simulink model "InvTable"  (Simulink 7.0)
settings: Solver=FixedStepDiscrete  StartTime=0.0  StopTime=inf  FixedStep=samplePeriod  RelTol=1e-3
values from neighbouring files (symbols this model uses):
  forceCanon = 0.00444822    [initialize.m]    (also in TableInit.m = 1)
  iactParams = [	actParams    [initialize.m]
  inertia = inertia + inertiaP2Q([0 0 0], massA(i), cgA(:,i)-cg,  									inertiaCanon, massCanon)    [initialize.m]    (also in TableInit.m = [Ixx 0 0; 0 Iyy 0; 0 0 Izz])
  inertiaMask = zeros(3, 1)    [initialize.m]
  initDispl = zeros(6, 1)    [initialize.m]
  lengthCanon = 25.4    [initialize.m]    (also in TableInit.m)
  mass = ones(3, 1) * (sum(massA) + massT + massS)    [initialize.m]    (also in TableInit.m = 17300)
  massMask = zeros(3, 1)    [initialize.m]
  returnPress = 50    [initialize.m]    (also in TableInit.m)
  rtg = cg    [initialize.m]    (also in TableInit.m = [0 0 cg])
  staticForce = forceT2A(ftbl, dtbl0, dof, rh, rb, rl, canon, atype)    [initialize.m]
undefined symbols (not defined in the file or in its folder): atype, friction, yieldDispl
libraries: LibTransforms x15, LibDynamics x12

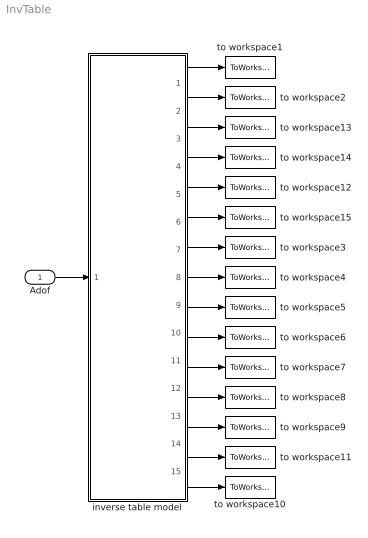
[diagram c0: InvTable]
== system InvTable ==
  Adof : Inport  PortDimensions=6  OutDataType=sfix(16)  OutScaling=2^0
  inverse table model : Subsystem
  to workspace1 : ToWorkspace  VariableName=xyz  SampleTime=-1  SaveFormat=Array
  to workspace10 : ToWorkspace  VariableName=svcmd  SampleTime=-1  SaveFormat=Array
  to workspace11 : ToWorkspace  VariableName=press  SampleTime=-1  SaveFormat=Array
  to workspace12 : ToWorkspace  VariableName=Axyz  SampleTime=-1  SaveFormat=Array
  to workspace13 : ToWorkspace  VariableName=Vxyz  SampleTime=-1  SaveFormat=Array
  to workspace14 : ToWorkspace  VariableName=Vrpw  SampleTime=-1  SaveFormat=Array
  to workspace15 : ToWorkspace  VariableName=Arpw  SampleTime=-1  SaveFormat=Array
  to workspace2 : ToWorkspace  VariableName=rpw  SampleTime=-1  SaveFormat=Array
  to workspace3 : ToWorkspace  VariableName=Fxyz  SampleTime=-1  SaveFormat=Array
  to workspace4 : ToWorkspace  VariableName=Frpw  SampleTime=-1  SaveFormat=Array
  to workspace5 : ToWorkspace  VariableName=Dact  SampleTime=-1  SaveFormat=Array
  to workspace6 : ToWorkspace  VariableName=Vact  SampleTime=-1  SaveFormat=Array
  to workspace7 : ToWorkspace  VariableName=Aact  SampleTime=-1  SaveFormat=Array
  to workspace8 : ToWorkspace  VariableName=Fact  SampleTime=-1  SaveFormat=Array
  to workspace9 : ToWorkspace  VariableName=flow  SampleTime=-1  SaveFormat=Array
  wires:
  inverse table model/1(xyz) -> to workspace1/1
  inverse table model/2(rpw) -> to workspace2/1
  inverse table model/7(Fxyz) -> to workspace3/1
  inverse table model/8(Frpw) -> to workspace4/1
  inverse table model/9(Dact) -> to workspace5/1
  inverse table model/10(Vact) -> to workspace6/1
  inverse table model/11(Aact) -> to workspace7/1
  inverse table model/12(Fact) -> to workspace8/1
  inverse table model/13(flow) -> to workspace9/1
  inverse table model/14(press) -> to workspace11/1
  Adof/1 -> inverse table model/1(Adof)
  inverse table model/15(svcmd) -> to workspace10/1
  inverse table model/3(Vxyz) -> to workspace13/1
  inverse table model/4(Vrpw) -> to workspace14/1
  inverse table model/5(Axyz) -> to workspace12/1
  inverse table model/6(Arpw) -> to workspace15/1

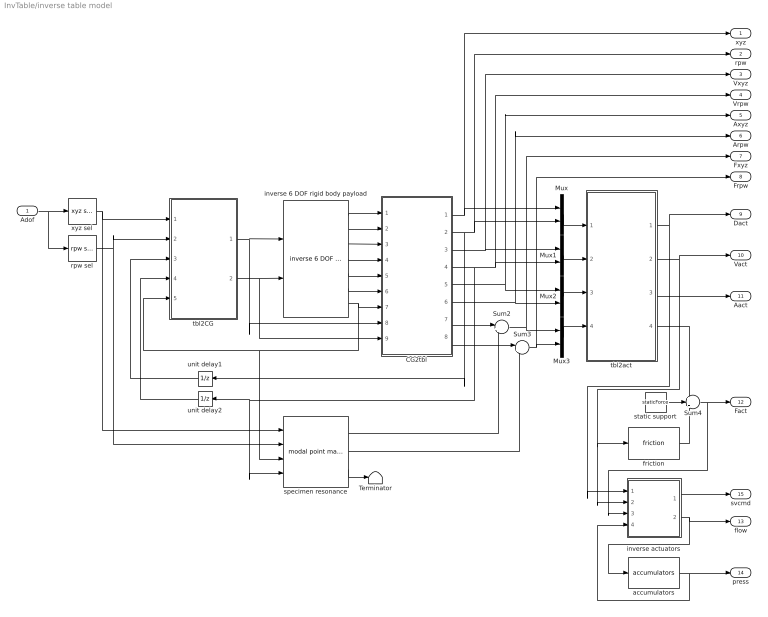
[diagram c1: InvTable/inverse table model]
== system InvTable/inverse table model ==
  Adof : Inport  PortDimensions=6  OutDataType=sfix(16)  OutScaling=2^0
  CG2tbl : Subsystem  mask{ofst=-rtg}
      mask prompts: ofst "Origin offset"
  Mux{,1..3} (4 alike) : Mux  Inputs=2
  Sum2 : Sum  Inputs=|++  OutDataType=sfix(16)  OutScaling=2^0
  Sum3 : Sum  Inputs=|++  OutDataType=sfix(16)  OutScaling=2^0
  Sum4 : Sum  Inputs=+-+  OutDataType=sfix(16)  OutScaling=2^0
  Terminator : Terminator
  accumulators : LibDynamics/accumulators  SystemSampleTime=-1  pumpFlow=pumpFlow  supplyPressure=supplyPress  precharge=precharge  bottleVolume=volume  gasConstant=gasConstant  flowCanon=flowCanon  volumeCanon=volumeCanon  samplePeriod=samplePeriod
  friction : LibDynamics/friction  SystemSampleTime=-1  friction=friction * forceCanon  yieldDispl=yieldDispl * lengthCanon  hysteresis=0  velocCanon=linVelocCanon  samplePeriod=samplePeriod
  inverse 6 DOF rigid body payload : LibDynamics/inverse 6 DOF rigid body payload  SystemSampleTime=-1  mass=mass.*massMask  inertia=diag(inertia.*inertiaMask)  gee=gee  massCanon=massCanon  inertiaCanon=inertiaCanon  linVelocCanon=linVelocCanon  linAccelCanon=linAccelCanon  rotDisplCanon=rotDisplCanon  rotVelocCanon=rotVelocCanon  rotAccelCanon=rotAccelCanon  rotForceCanon=rotForceCanon  initialPosition=initDispl  samplePeriod=samplePeriod
  inverse actuators : Subsystem
  rpw sel : LibTransforms/rpw sel  SystemSampleTime=-1  dof=1:6
  specimen resonance : LibDynamics/modal point mass  SystemSampleTime=-1  mass=modalMass  freq=modalFreq  damp=modalDamp  ofst=modalCG  gee=gee  massCanon=massCanon  linAccelCanon=linAccelCanon  rotDisplCanon=rotDisplCanon  rotVelocCanon=rotVelocCanon  rotForceCanon=rotForceCanon  samplePeriod=samplePeriod
  static support : Constant  Value=staticForce  OutDataType=sfix(16)  OutScaling=2^0
  tbl2CG : Subsystem  mask{ofst=rtg}
      mask prompts: ofst "Origin offset"
  tbl2act : Subsystem
  unit delay1 : UnitDelay  Orientation=left  X0=initDispl(4:6)  SampleTime=-1
  unit delay2 : UnitDelay  Orientation=left  SampleTime=-1
  xyz sel : LibTransforms/xyz sel  SystemSampleTime=-1  dof=1:6
  xyz : Outport  OutDataType=sfix(16)  OutScaling=2^0
  rpw : Outport  Port=2  OutDataType=sfix(16)  OutScaling=2^0
  Vxyz : Outport  Port=3  OutDataType=sfix(16)  OutScaling=2^0
  Vrpw : Outport  Port=4  OutDataType=sfix(16)  OutScaling=2^0
  Axyz : Outport  Port=5  OutDataType=sfix(16)  OutScaling=2^0
  Arpw : Outport  Port=6  OutDataType=sfix(16)  OutScaling=2^0
  Fxyz : Outport  Port=7  OutDataType=sfix(16)  OutScaling=2^0
  Frpw : Outport  Port=8  OutDataType=sfix(16)  OutScaling=2^0
  Dact : Outport  Port=9  OutDataType=sfix(16)  OutScaling=2^0
  Vact : Outport  Port=10  OutDataType=sfix(16)  OutScaling=2^0
  Aact : Outport  Port=11  OutDataType=sfix(16)  OutScaling=2^0
  Fact : Outport  Port=12  OutDataType=sfix(16)  OutScaling=2^0
  flow : Outport  Port=13  OutDataType=sfix(16)  OutScaling=2^0
  press : Outport  Port=14  OutDataType=sfix(16)  OutScaling=2^0
  svcmd : Outport  Port=15  OutDataType=sfix(16)  OutScaling=2^0
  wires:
  specimen resonance/3 -> Terminator/1
  static support/1 -> Sum4/2
  friction/1 -> Sum4/3
  Sum4/1 -> inverse actuators/3(force), Fact/1
  inverse actuators/2(flow) -> accumulators/1, flow/1
  xyz sel/1 -> tbl2CG/1(Axyz), specimen resonance/1
  accumulators/1 -> inverse actuators/4(press), press/1
  inverse actuators/1(cmd) -> svcmd/1
  tbl2CG/1(accel xyz) -> inverse 6 DOF rigid body payload/1, CG2tbl/8(accel xyz)
  rpw sel/1 -> tbl2CG/2(Arpw), specimen resonance/2
  tbl2CG/2(accel rpw) -> inverse 6 DOF rigid body payload/2, CG2tbl/9(accel rpw)
  CG2tbl/1(xyz) -> Mux/1, xyz/1
  CG2tbl/2(rpw) -> Mux/2, rpw/1, unit delay1/1
  CG2tbl/3(Vxyz) -> Mux1/1, Vxyz/1
  CG2tbl/4(Vrpw) -> Mux1/2, Vrpw/1, unit delay2/1, specimen resonance/4
  CG2tbl/5(Axyz) -> Mux2/1, Axyz/1
  CG2tbl/6(Arpw) -> Mux2/2, Arpw/1
  Mux/1 -> tbl2act/1(displT)
  Mux1/1 -> tbl2act/2(velocT)
  Mux2/1 -> tbl2act/3(accelT)
  Mux3/1 -> tbl2act/4(forceT)
  inverse 6 DOF rigid body payload/1 -> CG2tbl/1(displ xyz)
  inverse 6 DOF rigid body payload/2 -> CG2tbl/2(displ rpw)
  inverse 6 DOF rigid body payload/3 -> CG2tbl/3(veloc xyz)
  inverse 6 DOF rigid body payload/4 -> CG2tbl/4(veloc rpw)
  inverse 6 DOF rigid body payload/5 -> CG2tbl/5(force xyz)
  inverse 6 DOF rigid body payload/6 -> CG2tbl/6(force rpw)
  inverse 6 DOF rigid body payload/7 -> CG2tbl/7(DCM), tbl2CG/5(DCM), specimen resonance/3
  Adof/1 -> xyz sel/1, rpw sel/1
  tbl2act/1(displA) -> inverse actuators/1(displ), Dact/1
  tbl2act/2(velocA) -> friction/1, inverse actuators/2(veloc), Vact/1
  tbl2act/3(accelA) -> Aact/1
  tbl2act/4(forceA) -> Sum4/1
  unit delay2/1 -> tbl2CG/4(Vrpw)
  unit delay1/1 -> tbl2CG/3(rpw)
  Sum2/1 -> Mux3/1, Fxyz/1
  CG2tbl/7(Fxyz) -> Sum2/1
  CG2tbl/8(Frpw) -> Sum3/1
  Sum3/1 -> Mux3/2, Frpw/1
  specimen resonance/1 -> Sum2/2
  specimen resonance/2 -> Sum3/2

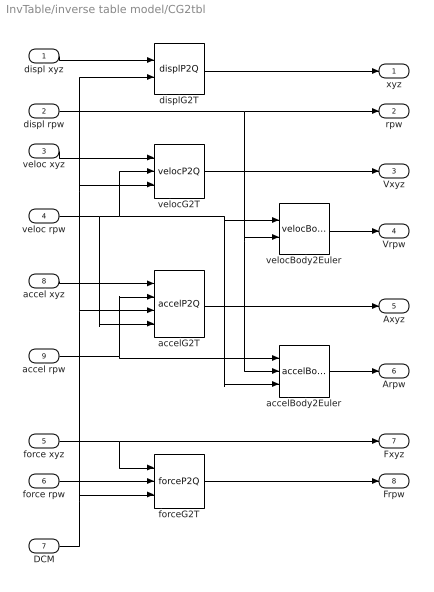
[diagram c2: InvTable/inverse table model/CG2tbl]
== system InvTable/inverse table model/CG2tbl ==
  displ xyz : Inport  OutDataType=sfix(16)  OutScaling=2^0
  displ rpw : Inport  Port=2  OutDataType=sfix(16)  OutScaling=2^0
  veloc xyz : Inport  Port=3  OutDataType=sfix(16)  OutScaling=2^0
  veloc rpw : Inport  Port=4  OutDataType=sfix(16)  OutScaling=2^0
  force xyz : Inport  Port=5  OutDataType=sfix(16)  OutScaling=2^0
  force rpw : Inport  Port=6  OutDataType=sfix(16)  OutScaling=2^0
  DCM : Inport  Port=7  OutDataType=sfix(16)  OutScaling=2^0
  accel xyz : Inport  Port=8  OutDataType=sfix(16)  OutScaling=2^0
  accel rpw : Inport  Port=9  OutDataType=sfix(16)  OutScaling=2^0
  accelBody2Euler : LibTransforms/accelBody2Euler  SystemSampleTime=-1  dof=1:6
  accelG2T : LibTransforms/accelP2Q  SystemSampleTime=-1  dof=1:6  ofst=ofst
  displG2T : LibTransforms/displP2Q  SystemSampleTime=-1  dof=1:6  ofst=ofst
  forceG2T : LibTransforms/forceP2Q  SystemSampleTime=-1  dof=1:6  ofst=ofst
  velocBody2Euler : LibTransforms/velocBody2Euler  SystemSampleTime=-1  dof=1:6
  velocG2T : LibTransforms/velocP2Q  SystemSampleTime=-1  dof=1:6  ofst=ofst
  xyz : Outport  OutDataType=sfix(16)  OutScaling=2^0
  rpw : Outport  Port=2  OutDataType=sfix(16)  OutScaling=2^0
  Vxyz : Outport  Port=3  OutDataType=sfix(16)  OutScaling=2^0
  Vrpw : Outport  Port=4  OutDataType=sfix(16)  OutScaling=2^0
  Axyz : Outport  Port=5  OutDataType=sfix(16)  OutScaling=2^0
  Arpw : Outport  Port=6  OutDataType=sfix(16)  OutScaling=2^0
  Fxyz : Outport  Port=7  OutDataType=sfix(16)  OutScaling=2^0
  Frpw : Outport  Port=8  OutDataType=sfix(16)  OutScaling=2^0
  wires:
  displ xyz/1 -> displG2T/1
  displG2T/1 -> xyz/1
  displ rpw/1 -> rpw/1, accelBody2Euler/2, velocBody2Euler/2
  veloc xyz/1 -> velocG2T/1
  velocBody2Euler/1 -> Vrpw/1
  veloc rpw/1 -> velocG2T/2, velocBody2Euler/1, accelBody2Euler/3, accelG2T/4
  velocG2T/1 -> Vxyz/1
  force xyz/1 -> forceG2T/1, Fxyz/1
  force rpw/1 -> forceG2T/2
  accel xyz/1 -> accelG2T/1
  accelG2T/1 -> Axyz/1
  accel rpw/1 -> accelBody2Euler/1, accelG2T/2
  accelBody2Euler/1 -> Arpw/1
  forceG2T/1 -> Frpw/1
  DCM/1 -> displG2T/2, velocG2T/3, accelG2T/3, forceG2T/3

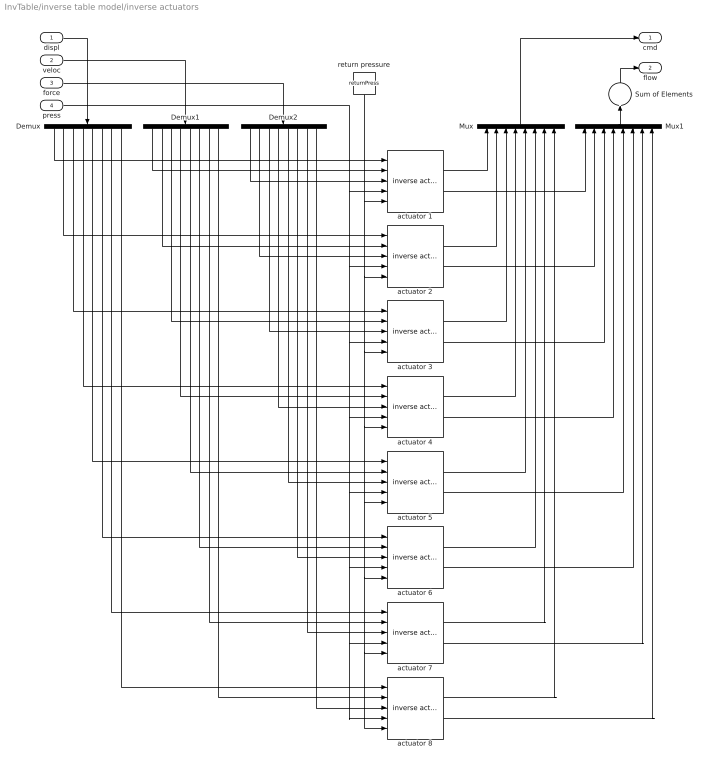
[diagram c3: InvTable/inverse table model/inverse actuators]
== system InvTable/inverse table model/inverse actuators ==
  displ : Inport  OutDataType=sfix(16)  OutScaling=2^0
  veloc : Inport  Port=2  OutDataType=sfix(16)  OutScaling=2^0
  force : Inport  Port=3  OutDataType=sfix(16)  OutScaling=2^0
  press : Inport  Port=4  OutDataType=sfix(16)  OutScaling=2^0
  Demux : Demux  Orientation=down  Outputs=nAct
  Demux1 : Demux  Orientation=down  Outputs=nAct
  Demux2 : Demux  Orientation=down  Outputs=nAct
  Mux : Mux  Orientation=up  Inputs=nAct
  Mux1 : Mux  Orientation=up  Inputs=nAct
  Sum of Elements : Sum  Orientation=up  Inputs=+  OutDataType=sfix(16)  OutScaling=2^-10
  actuator 1 : LibDynamics/inverse actuator  SystemSampleTime=-1  params=iactParams(:,1)
  actuator 2 : LibDynamics/inverse actuator  SystemSampleTime=-1  params=iactParams(:,2)
  actuator 3 : LibDynamics/inverse actuator  SystemSampleTime=-1  params=iactParams(:,3)
  actuator 4 : LibDynamics/inverse actuator  SystemSampleTime=-1  params=iactParams(:,4)
  actuator 5 : LibDynamics/inverse actuator  SystemSampleTime=-1  params=iactParams(:,5)
  actuator 6 : LibDynamics/inverse actuator  SystemSampleTime=-1  params=iactParams(:,6)
  actuator 7 : LibDynamics/inverse actuator  SystemSampleTime=-1  params=iactParams(:,7)
  actuator 8 : LibDynamics/inverse actuator  SystemSampleTime=-1  params=iactParams(:,8)
  return pressure : Constant  Orientation=down  Value=returnPress  OutDataType=sfix(16)  OutScaling=2^0
  cmd : Outport  OutDataType=sfix(16)  OutScaling=2^0
  flow : Outport  Port=2  OutDataType=sfix(16)  OutScaling=2^0
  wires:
  force/1 -> Demux2/1
  Mux/1 -> cmd/1
  Sum of Elements/1 -> flow/1
  return pressure/1 -> actuator 1/5, actuator 2/5, actuator 3/5, actuator 4/5, actuator 5/5, actuator 6/5, actuator 8/5, actuator 7/5
  press/1 -> actuator 1/4, actuator 2/4, actuator 3/4, actuator 4/4, actuator 5/4, actuator 6/4, actuator 8/4, actuator 7/4
  Mux1/1 -> Sum of Elements/1
  actuator 8/2 -> Mux1/8
  actuator 7/2 -> Mux1/7
  actuator 6/2 -> Mux1/6
  actuator 5/2 -> Mux1/5
  actuator 4/2 -> Mux1/4
  actuator 3/2 -> Mux1/3
  actuator 2/2 -> Mux1/2
  actuator 1/2 -> Mux1/1
  actuator 2/1 -> Mux/2
  actuator 1/1 -> Mux/1
  actuator 8/1 -> Mux/8
  actuator 7/1 -> Mux/7
  actuator 6/1 -> Mux/6
  actuator 5/1 -> Mux/5
  actuator 4/1 -> Mux/4
  actuator 3/1 -> Mux/3
  Demux2/8 -> actuator 8/3
  Demux1/8 -> actuator 8/2
  Demux/8 -> actuator 8/1
  Demux2/7 -> actuator 7/3
  Demux1/7 -> actuator 7/2
  Demux/7 -> actuator 7/1
  Demux2/6 -> actuator 6/3
  Demux1/6 -> actuator 6/2
  Demux/6 -> actuator 6/1
  Demux2/5 -> actuator 5/3
  Demux1/5 -> actuator 5/2
  Demux/5 -> actuator 5/1
  Demux2/4 -> actuator 4/3
  Demux1/4 -> actuator 4/2
  Demux/4 -> actuator 4/1
  Demux2/3 -> actuator 3/3
  Demux1/3 -> actuator 3/2
  Demux/3 -> actuator 3/1
  Demux2/2 -> actuator 2/3
  Demux1/2 -> actuator 2/2
  Demux2/1 -> actuator 1/3
  Demux1/1 -> actuator 1/2
  Demux/2 -> actuator 2/1
  Demux/1 -> actuator 1/1
  veloc/1 -> Demux1/1
  displ/1 -> Demux/1

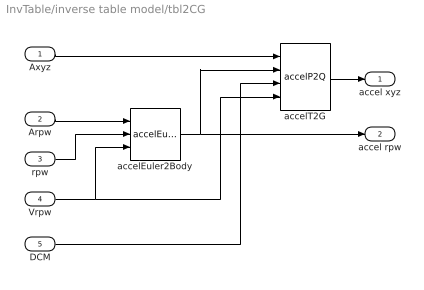
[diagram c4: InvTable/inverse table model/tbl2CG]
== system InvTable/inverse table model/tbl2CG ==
  Axyz : Inport  OutDataType=sfix(16)  OutScaling=2^0
  Arpw : Inport  Port=2  OutDataType=sfix(16)  OutScaling=2^0
  rpw : Inport  Port=3  OutDataType=sfix(16)  OutScaling=2^0
  Vrpw : Inport  Port=4  OutDataType=sfix(16)  OutScaling=2^0
  DCM : Inport  Port=5  OutDataType=sfix(16)  OutScaling=2^0
  accelEuler2Body : LibTransforms/accelEuler2Body  SystemSampleTime=-1  dof=1:6
  accelT2G : LibTransforms/accelP2Q  SystemSampleTime=-1  dof=1:6  ofst=ofst
  accel xyz : Outport  OutDataType=sfix(16)  OutScaling=2^0
  accel rpw : Outport  Port=2  OutDataType=sfix(16)  OutScaling=2^0
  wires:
  Axyz/1 -> accelT2G/1
  accelT2G/1 -> accel xyz/1
  Arpw/1 -> accelEuler2Body/1
  accelEuler2Body/1 -> accelT2G/2, accel rpw/1
  Vrpw/1 -> accelT2G/4, accelEuler2Body/3
  rpw/1 -> accelEuler2Body/2
  DCM/1 -> accelT2G/3

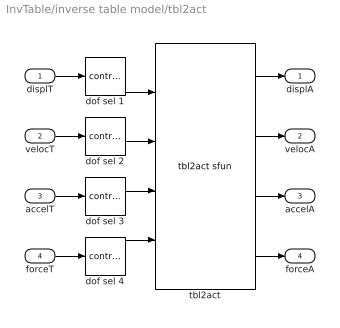
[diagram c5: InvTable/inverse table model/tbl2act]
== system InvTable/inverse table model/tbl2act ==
  displT : Inport
  velocT : Inport  Port=2
  accelT : Inport  Port=3
  forceT : Inport  Port=4
  dof sel {1..4} (4 alike) : LibTransforms/contract  SystemSampleTime=-1  elements=dof
  tbl2act : LibTransforms/tbl2act sfun  atype=atype  nVel=length(atype)  nFrc=length(atype)  dof=dof  rh=rh  rb=rb  rl=rl  ra=ra  ea=ea  offset=[0 0 0 0 0 0]  fmax=fmax  canon=canon  gee=gee  action=1  rate=0
  displA : Outport
  velocA : Outport  Port=2
  accelA : Outport  Port=3
  forceA : Outport  Port=4
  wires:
  dof sel 4/1 -> tbl2act/4
  dof sel 3/1 -> tbl2act/3
  dof sel 2/1 -> tbl2act/2
  dof sel 1/1 -> tbl2act/1
  tbl2act/4 -> forceA/1
  forceT/1 -> dof sel 4/1
  tbl2act/3 -> accelA/1
  accelT/1 -> dof sel 3/1
  tbl2act/2 -> velocA/1
  velocT/1 -> dof sel 2/1
  tbl2act/1 -> displA/1
  displT/1 -> dof sel 1/1
